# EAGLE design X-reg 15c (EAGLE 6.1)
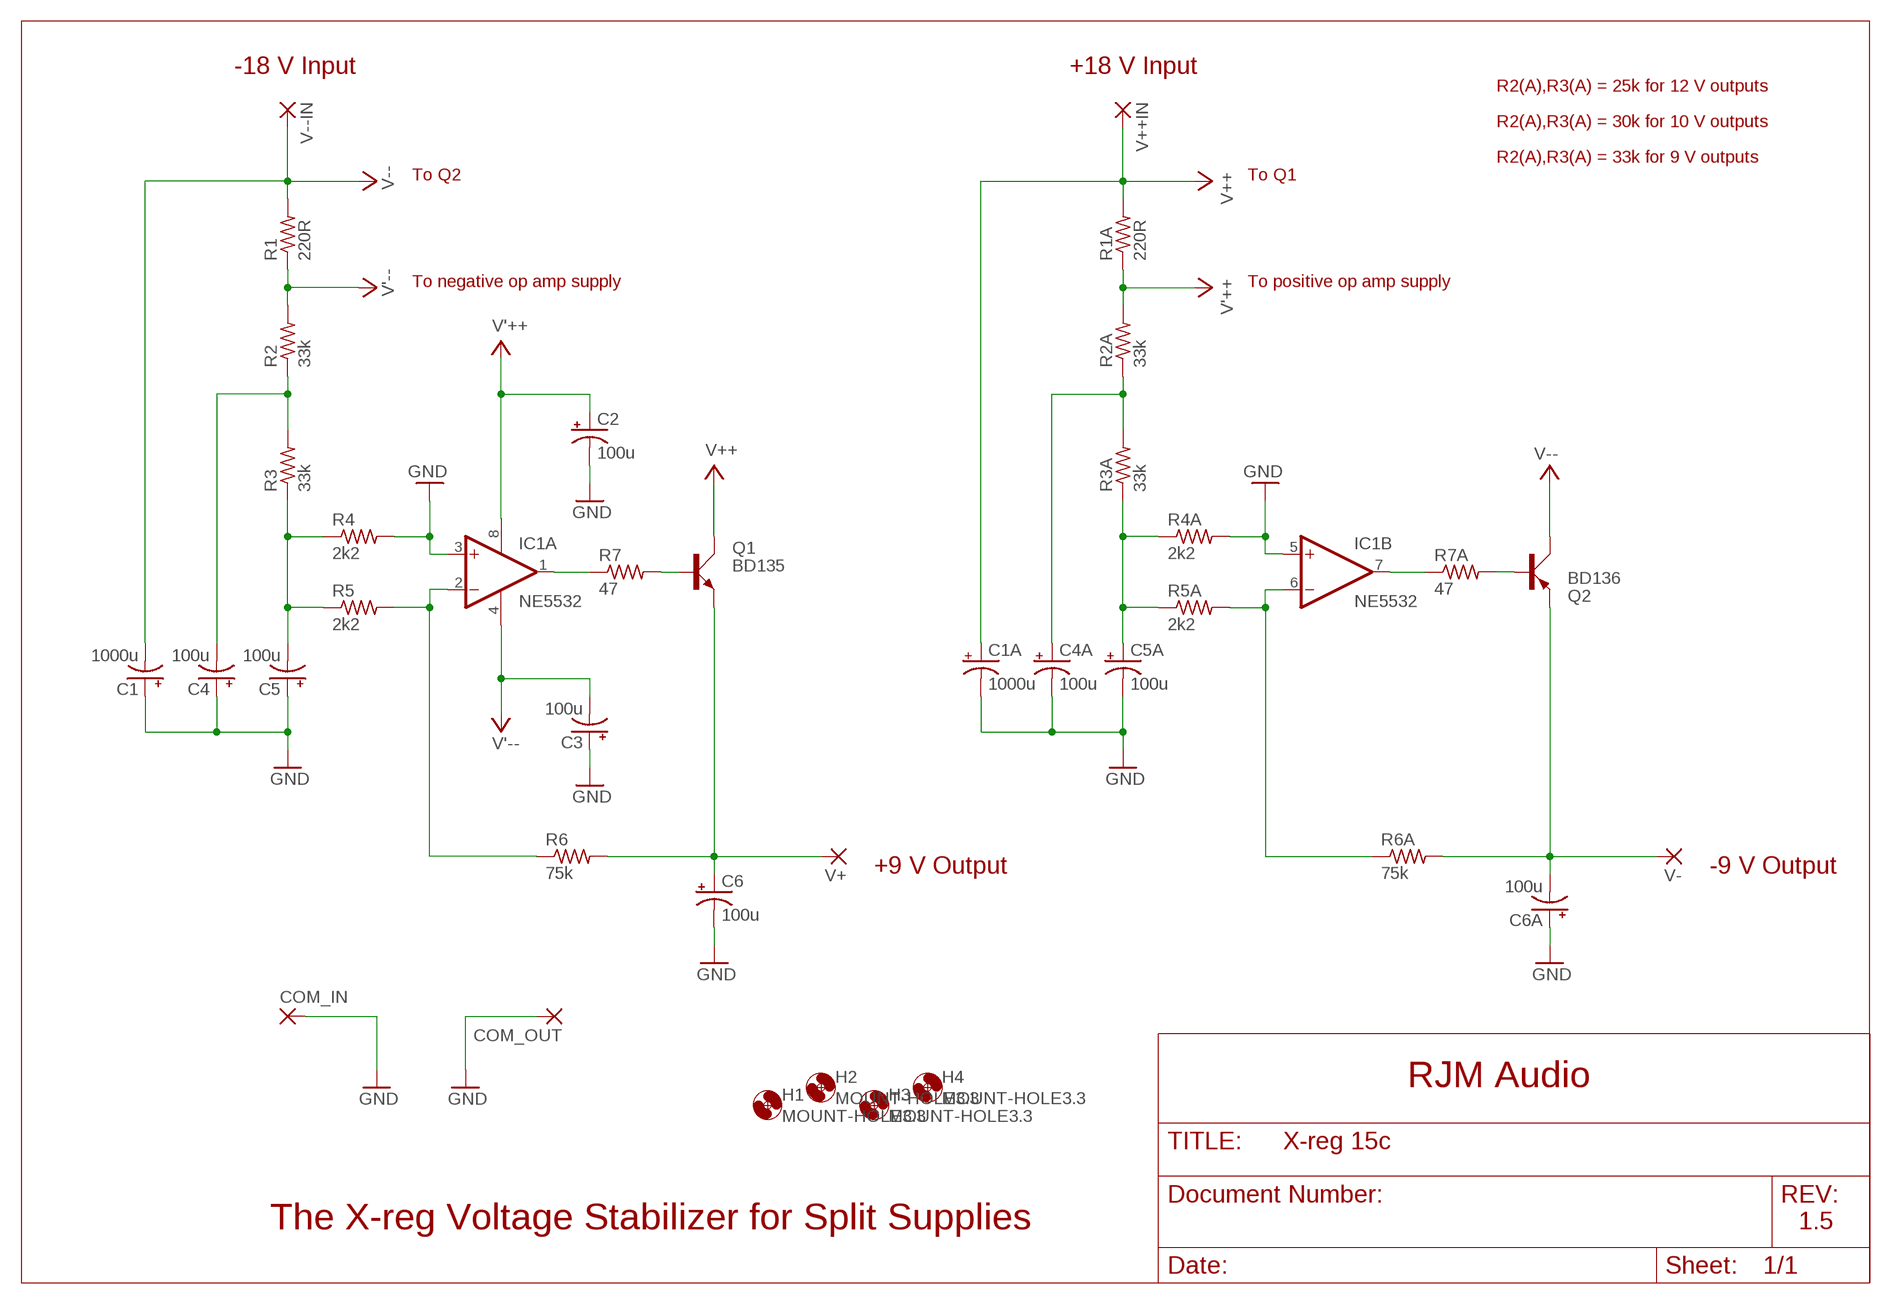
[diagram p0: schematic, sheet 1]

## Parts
C1  1000u  CPOL-USE5-10.5  [E5-10,5]
C1A  1000u  CPOL-USE5-10.5  [E5-10,5]
C2  100u  CPOL-USE2.5-6  [E2,5-6]
C3  100u  CPOL-USE2.5-6  [E2,5-6]
C4  100u  CPOL-USE2.5-6  [E2,5-6]
C4A  100u  CPOL-USE2.5-6  [E2,5-6]
C5  100u  CPOL-USE2.5-6  [E2,5-6]
C5A  100u  CPOL-USE2.5-6  [E2,5-6]
C6  100u  CPOL-USE2.5-6  [E2,5-6]
C6A  100u  CPOL-USE2.5-6  [E2,5-6]
COM_IN  3,17/1,3  [3,17/1,3]
COM_OUT  3,17/1,3  [3,17/1,3]
H1  MOUNT-HOLE3.3  [3,3]
H2  MOUNT-HOLE3.3  [3,3]
H3  MOUNT-HOLE3.3  [3,3]
H4  MOUNT-HOLE3.3  [3,3]
IC1  NE5532  OPA2344P  [DIL08]
Q1  BD135  BD139  [TO126AV]
Q2  BD136  BD140  [TO126AV]
R1  220R  R-US_0207/10  [0207/10]
R1A  220R  R-US_0207/10  [0207/10]
R2  33k  R-US_0207/10  [0207/10]
R2A  33k  R-US_0207/10  [0207/10]
R3  33k  R-US_0207/10  [0207/10]
R3A  33k  R-US_0207/10  [0207/10]
R4  2k2  R-US_0207/10  [0207/10]
R4A  2k2  R-US_0207/10  [0207/10]
R5  2k2  R-US_0207/10  [0207/10]
R5A  2k2  R-US_0207/10  [0207/10]
R6  75k  R-US_0207/10  [0207/10]
R6A  75k  R-US_0207/10  [0207/10]
R7  47  R-US_0207/10  [0207/10]
R7A  47  R-US_0207/10  [0207/10]
V+  3,17/1,3  [3,17/1,3]
V++IN  3,17/1,3  [3,17/1,3]
V-  3,17/1,3  [3,17/1,3]
V--IN  3,17/1,3  [3,17/1,3]

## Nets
GND: C1.+ C1A.- C2.- C3.+ C4.+ C4A.- C5.+ C5A.- C6.- C6A.+ COM_IN.1(P) COM_OUT.1(P) IC1.3(A:+IN) IC1.5(B:+IN) R4.2 R4A.2
N$2: IC1.1(A:OUT) R7.1
N$3: Q1.B R7.2
N$4: IC1.7(B:OUT) R7A.1
N$5: Q2.B R7A.2
V'++: C2.+ IC1.8(A:V+) R1A.1 R2A.2
V'--: C3.- IC1.4(A:V-) R1.1 R2.2
V+: C6.+ Q1.E R6.2 V+.1(P)
V++: C1A.+ Q1.C R1A.2 V++IN.1(P)
V+FILTER: C4A.+ R2A.1 R3A.2
V+INV: IC1.6(B:-IN) R5A.2 R6A.1
V+REF: C5A.+ R3A.1 R4A.1 R5A.1
V-: C6A.- Q2.E R6A.2 V-.1(P)
V--: C1.- Q2.C R1.2 V--IN.1(P)
V-FILTER: C4.- R2.1 R3.2
V-INV: IC1.2(A:-IN) R5.2 R6.1
V-REF: C5.- R3.1 R4.1 R5.1

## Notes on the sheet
- -18 V Input | +18 V Input
- R2(A),R3(A) = 25k for 12 V outputs
- R2(A),R3(A) = 30k for 10 V outputs
- R2(A),R3(A) = 33k for 9 V outputs
- To Q2 | To Q1
- To negative op amp supply | To positive op amp supply
- +9 V Output | -9 V Output
- RJM Audio
- The X-reg Voltage Stabilizer for Split Supplies | 1.5

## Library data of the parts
C1 C1A = resistor:CPOL-US: POLARIZED CAPACITOR, American symbol
C2-C4 C4A C5 C5A C6 C6A = rcl:CPOL-US: POLARIZED CAPACITOR, American symbol
COM_IN COM_OUT V+ V++IN V- V--IN = wirepad:3,17/1,3: THROUGH-HOLE PAD
H1-H4 = holes:MOUNT-HOLE: MOUNTING HOLE with drill center marker
IC1 = linear:OPA2*: Dual Operational Amplifier Low Power, Single-Supply, Rail-To-Rail Operational Amplifier Source: http://focus.ti.com/lit/ds/symlink/opa2345.pdf http://focus.ti.com .. opa241.pdf http://focus.ti.com/lit/ds/symlink/opa2134.pdf
Q1 = transistor-power:BD139: NPN TRANSISTOR
Q2 = transistor-power:BD140: PNP TRANSISTOR
R1 R1A R2 R2A R3 R3A R4 R4A R5 R5A R6 R6A R7 R7A = rcl:R-US_: RESISTOR, American symbol

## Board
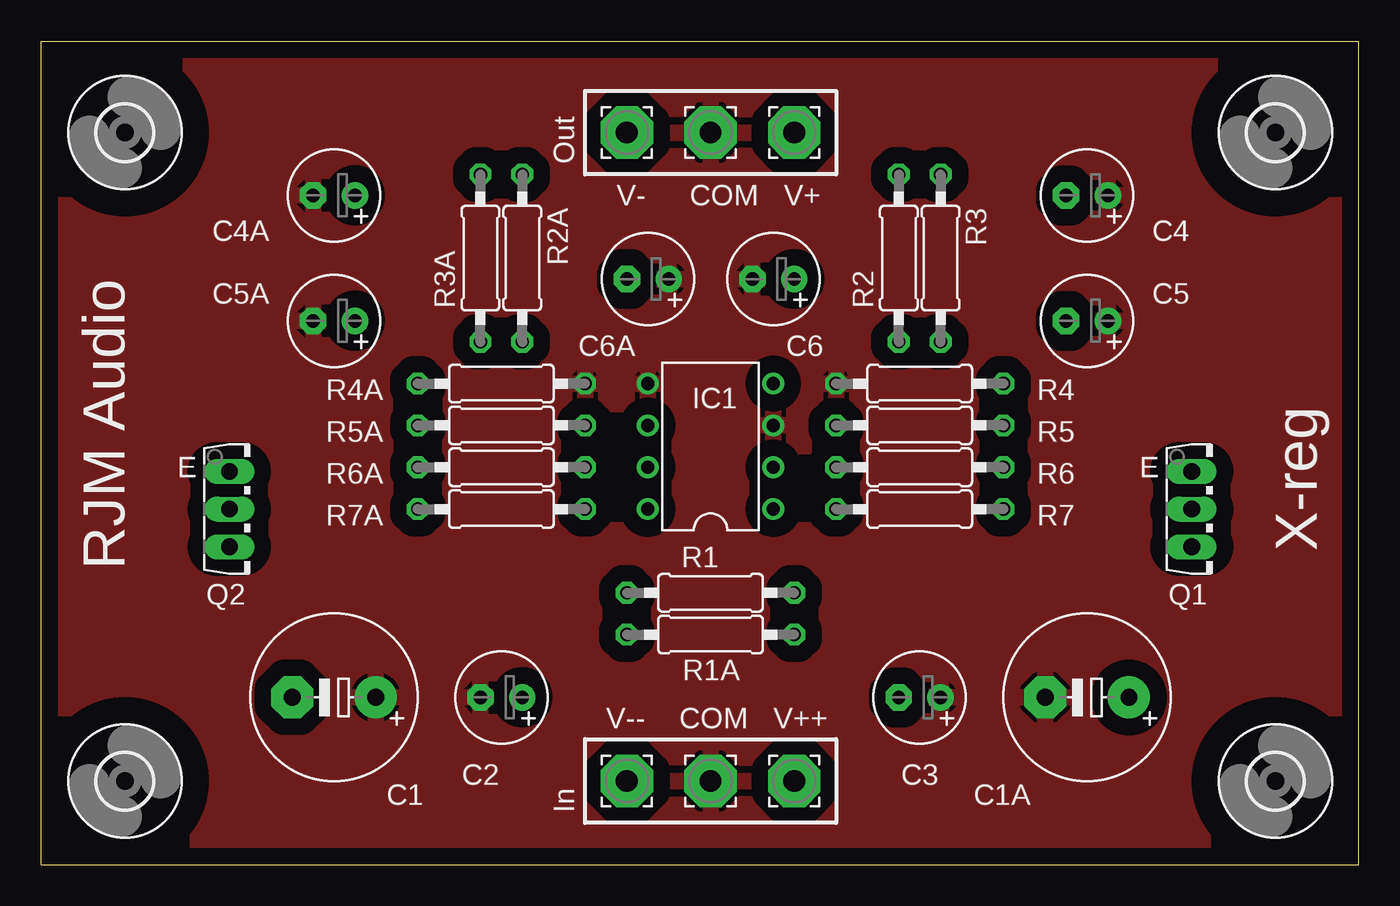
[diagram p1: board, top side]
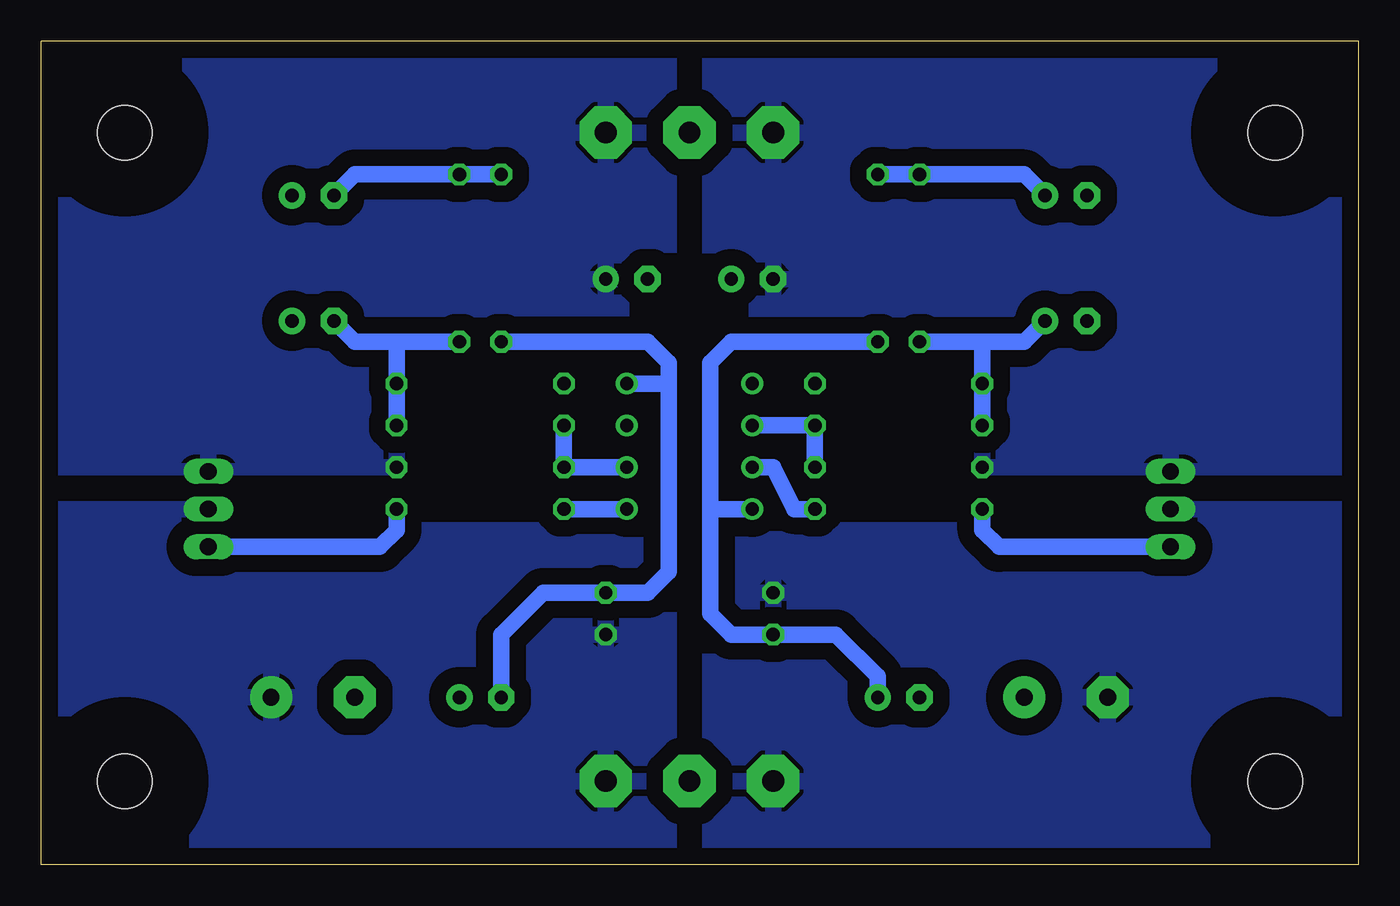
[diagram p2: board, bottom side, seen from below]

Size 80 x 50 mm. Coordinates in mm from the lower left corner, seen from the top.
Outline: 0,0 80,0 80,50 0,50 0,0
Copper layers (1*16): Top 0.035mm / dielectric 1.5mm / Bottom 0.035mm
Design rules: minimum track width 10mil, minimum drill 24mil, track to track 8mil, track to pad 8mil, pad to pad 8mil, via to via 8mil, smd to smd 8mil, copper to edge 40mil, drill to drill 8mil, minimum pad ring 10mil, minimum via ring 8mil, stop-mask expansion 4mil, vias tented up to drill 0mil, thermal gap 10mil

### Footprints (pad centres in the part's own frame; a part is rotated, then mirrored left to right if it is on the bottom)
E5-10,5 = drill 1.016 pad 2.54: + -2.54,0 | drill 1.016 pad 2.54 octagon: - 2.54,0
E2,5-6 = drill 0.813 pad 1.6: + -1.27,0 | drill 0.813 pad 1.6 octagon: - 1.27,0
3,17/1,3 = drill 1.321 pad 3.175 octagon: 1 0,0
3,3 = hole 3.3: 0,0
DIL08 = drill 0.813 pad 1.27: 1 -3.81,-3.81; 2 -1.27,-3.81; 3 1.27,-3.81; 4 3.81,-3.81; 5 3.81,3.81; 6 1.27,3.81; 7 -1.27,3.81; 8 -3.81,3.81
TO126AV = drill 1.016 long: B 2.286,-1.27; C 0,-1.27; E -2.286,-1.27
0207/10 = drill 0.813 octagon: 1 -5.08,0; 2 5.08,0

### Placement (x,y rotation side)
C1  17.78,10.16 180 top
C1A  63.5,10.16 180 top
C2  27.94,10.16 180 top
C3  53.34,10.16 180 top
C4  63.5,40.64 180 top
C4A  17.78,40.64 180 top
C5  63.5,33.02 180 top
C5A  17.78,33.02 180 top
C6  44.45,35.56 180 top
C6A  36.83,35.56 180 top
COM_IN  40.64,5.08 0 top
COM_OUT  40.64,44.45 0 top
H1  5.08,5.08 0 top
H2  5.08,44.45 0 top
H3  74.93,44.45 0 top
H4  74.93,5.08 0 top
IC1  40.64,25.4 90 top
Q1  71.12,21.59 270 top
Q2  12.7,21.59 270 top
R1  40.64,16.51 180 top
R1A  40.64,13.97 0 top
R2  52.07,36.83 270 top
R2A  29.21,36.83 270 top
R3  54.61,36.83 90 top
R3A  26.67,36.83 90 top
R4  53.34,29.21 180 top
R4A  27.94,29.21 0 top
R5  53.34,26.67 180 top
R5A  27.94,26.67 0 top
R6  53.34,24.13 0 top
R6A  27.94,24.13 180 top
R7  53.34,21.59 0 top
R7A  27.94,21.59 180 top
V+  45.72,44.45 0 top
V++IN  45.72,5.08 0 top
V-  35.56,44.45 0 top
V--IN  35.56,5.08 0 top

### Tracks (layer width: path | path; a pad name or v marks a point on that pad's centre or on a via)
GND
  pour Top (isolate 1.016): 0,50.8 80.01,50.8 80.01,0 0,0
N$2
  Bottom 1.016: IC1.1 R7.1
N$3
  Bottom 1.016: Q1.B 59.44,19.3 58.42,20.32 R7.2
N$4
  Bottom 1.016: IC1.7 35.56,24.13 34.29,21.59 R7A.1
N$5
  Bottom 1.016: Q2.B 21.84,19.3 22.86,20.32 R7A.2
V'++
  Bottom 1.016: 39.37,21.59 39.37,15.24 38.1,13.97 R1A.1 31.75,13.97 29.21,11.43 C2.+ | 39.37,21.59 39.37,30.48 38.1,31.75 R2A.2 | IC1.8 39.37,21.59
V'--
  Bottom 1.016: 41.91,29.21 41.91,17.78 43.18,16.51 R1.1 49.53,16.51 52.07,13.97 C3.- | 41.91,29.21 41.91,30.48 43.18,31.75 R2.2 | IC1.4 41.91,29.21
V+
  pour Bottom (isolate 1.016): 41.91,50.8 80.01,50.8 80.01,24.13 58.42,24.13 58.42,31.75 41.91,31.75
V++
  pour Bottom (isolate 1.016): 41.91,0 41.91,20.32 69.85,20.32 69.85,21.59 80.01,21.59 80.01,0
V+FILTER
  Bottom 1.016: C4A.+ 20.32,41.91 R3A.2 R2A.1
V+INV
  Bottom 1.016: IC1.6 R5A.2 R6A.1
V+REF
  Bottom 1.016: R3A.1 22.86,31.75 | 22.86,31.75 20.32,31.75 C5A.+ | 22.86,31.75 R4A.1 R5A.1
V-
  pour Bottom (isolate 1.016): 0,24.13 22.86,24.13 22.86,31.75 39.37,31.75 39.37,50.8 0,50.8
V--
  pour Bottom (isolate 1.016): 0,0 39.37,0 39.37,20.32 11.43,20.32 11.43,21.59 0,21.59
V-FILTER
  Bottom 1.016: C4.- 60.96,41.91 R3.2 R2.1
V-INV
  Bottom 1.016: R5.2 R6.1 IC1.2
V-REF
  Bottom 1.016: C5.- 60.96,31.75 58.42,31.75 | 58.42,31.75 R3.1 | R5.1 R4.1 58.42,31.75

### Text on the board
tPlace: Out | V- | COM | V+ | RJM Audio | E | E | X-reg | V-- | COM | V++ | In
